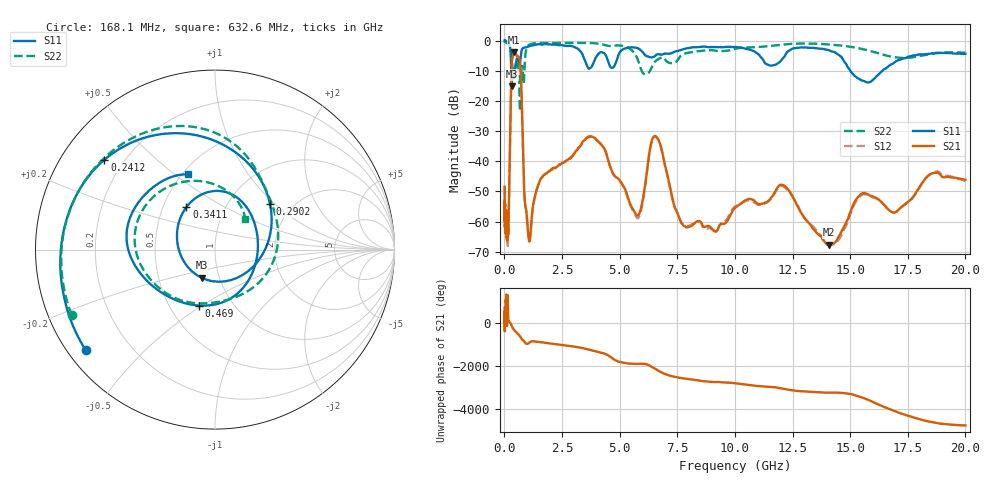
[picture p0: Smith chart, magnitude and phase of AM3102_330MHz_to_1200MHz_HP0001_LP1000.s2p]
! Date/Time: Tue, Sep 11, 2018 5:09 PM
! Network Analyzer: Agilent Technologies E8362B Rev: A.07.50.63
! Sweep from 0.010 to 20.000 GHz, 1601 Points, Sweep Type: LOG
! Power Supply: 4.950 V, 0.001 A
# Hz S DB R 50
!freq MagS11 AngS11 MagS21 AngS21 MagS12 AngS12 MagS22 AngS22
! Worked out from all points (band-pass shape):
!   1601 points, 10 MHz to 20 GHz, reference 50 ohm
!   highest |S21| = -3.84 dB at 432.6 MHz (marker M1); lowest = -67.7 dB at 14.07 GHz (marker M2)
!   |S21| within 3 dB of the highest: 328.1 MHz to 673.9 MHz (345.8 MHz wide, 69 % of centre)
!   lowest |S11| = -15.2 dB at 316.2 MHz (marker M3), VSWR 1.42, Z = 41.1 - j13.3 ohm
!   |S11| at or under -10 dB: 296.1 MHz to 349.9 MHz (53.83 MHz wide, 16.7 % of centre); 370.8 MHz to 464.7 MHz (93.92 MHz wide, 22.5 % of centre); 15.01 GHz to 16.4 GHz (1.395 GHz wide, 8.88 % of centre)
!   |S22| runs from -23.4 to -0.3 dB; largest |S21 - S12| = 0.012
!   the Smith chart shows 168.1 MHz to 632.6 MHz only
!   S11 on the Smith chart (normalised r, x): 168.1 MHz: 0.05, -0.34; 241.2 MHz: 0.13, +0.35; 290.2 MHz: 1.55, +0.93; 341.1 MHz: 0.66, +0.34; 469 MHz: 0.70, -0.49; 632.6 MHz: 0.54, +0.56
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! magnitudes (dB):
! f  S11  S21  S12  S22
! 10 MHz  0.0  -48.4  -48.3  -0.3
! 35.55 MHz  0.0  -59.8  -61.0  -0.5
! 126.4 MHz  -0.4  -65.5  -64.4  -0.9
! 168.1 MHz  -0.8  -63.7  -61.3  -1.1
! 241.2 MHz  -2.0  -35.2  -35.2  -1.8
! 290.2 MHz  -8.0  -14.6  -14.7  -3.7
! 316.2 MHz  -15.2  -8.2  -8.2  -6.3
! 341.1 MHz  -10.9  -6.0  -6.0  -8.2
! 432.6 MHz  -11.7  -3.8  -3.9  -10.0
! 447.2 MHz  -10.9  -3.9  -3.9  -9.4
! 469 MHz  -9.8  -4.0  -4.0  -8.6
! 632.6 MHz  -7.0  -5.6  -5.7  -12.3
! 682.6 MHz  -7.2  -7.4  -7.5  -23.3
! 1.057 GHz  -1.9  -65.5  -65.9  -1.5
! 1.59 GHz  -1.3  -45.7  -45.7  -0.8
! 3.793 GHz  -8.6  -31.8  -31.7  -0.9
! 5.652 GHz  -2.3  -56.8  -57.5  -4.3
! 6.58 GHz  -4.8  -31.8  -32.0  -6.6
! 7.845 GHz  -2.7  -61.6  -61.3  -4.3
! 12.09 GHz  -5.9  -47.9  -48.3  -1.3
! 14.07 GHz  -3.2  -67.7  -67.6  -1.3
! 20 GHz  -4.4  -46.1  -46.6  -4.0
